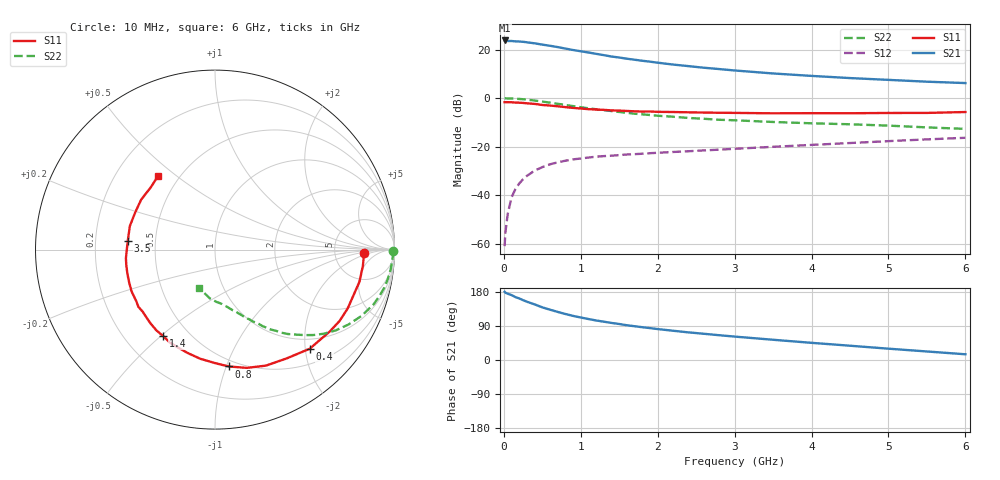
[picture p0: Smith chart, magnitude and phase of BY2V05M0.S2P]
! SIEMENS Small Signal Semiconductors
! BFY420
! Si NPN RF SIEGET Grounded Emitter Transistor in MICRO-X
! VCE = 2 V  IC = 5 mA
! Common Emitter S-Parameters:  October  1996
# GHz  S  MA  R  50
!  f  S11  S21  S12  S22
! GHz  MAG  ANG  MAG  ANG  MAG  ANG  MAG  ANG
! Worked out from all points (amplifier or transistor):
!   36 points, 10 MHz to 6 GHz, reference 50 ohm
!   highest |S21| = 23.8 dB at 10 MHz (marker M1)
!   |S21| within 3 dB of that: start of sweep to 743.9 MHz
!   unconditionally stable (mu >= 1): 3.149 GHz to end of sweep
!   at 250 MHz: K = 0.11, MSG = 28.3 dB, |S12| = -33.4 dB
!   at 1.4 GHz: K = 0.53, MSG = 20.4 dB, |S12| = -23.7 dB
!   at 6 GHz: K = 1.14, MAG = 9.0 dB, |S12| = -16.3 dB
!   S11 on the Smith chart (normalised r, x): 10 MHz: 10, -1; 400 MHz: 0.79, -2.09; 800 MHz: 0.45, -1.02; 1.4 GHz: 0.36, -0.51; 3.5 GHz: 0.34, +0.04; 6 GHz: 0.38, +0.43
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0.01  0.8283 -1.4  15.45 180.0  0.0009 110.8  0.9908 -0.5
0.02  0.8297 -2.6  15.36 177.6  0.0017 81.7  0.9938 -1.3
0.05  0.829 -6.2  15.06 174.9  0.0041 88.1  0.9894 -3.1
0.1  0.8247 -12.5  15.06 171.3  0.0091 85.3  0.985 -6.5
0.15  0.8129 -18.0  14.8 166.0  0.0134 78.6  0.9762 -9.8
0.2  0.8088 -23.9  14.7 162.5  0.0175 78.4  0.9666 -12.7
0.3  0.7855 -35.5  14.16 153.8  0.0252 71.8  0.9356 -18.9
0.4  0.7639 -46.3  13.49 146.8  0.0323 66.4  0.8966 -24.3
0.5  0.726 -56.6  12.68 138.9  0.0381 61.9  0.8528 -29.3
0.6  0.706 -66.3  12.02 132.8  0.0436 57.7  0.8103 -33.7
0.7  0.6826 -74.9  11.28 126.9  0.0478 54.3  0.7677 -37.6
0.8  0.6557 -83.3  10.51 121.4  0.0517 50.8  0.7257 -41.0
0.9  0.6316 -90.2  9.829 116.4  0.0551 48.2  0.6881 -43.8
1.1  0.596 -104.7  8.734 108.1  0.0601 44.4  0.6212 -49.2
1.4  0.5612 -121.1  7.213 97.8  0.0656 40.3  0.5443 -55.0
1.8  0.5309 -139.3  5.901 86.5  0.072 37.2  0.4655 -60.8
2.2  0.5199 -153.4  4.928 77.2  0.0782 35.6  0.4157 -65.8
2.8  0.502 -169.8  3.979 65.4  0.0874 34.1  0.36 -72.0
3.5  0.4886 174.5  3.232 53.4  0.0999 32.5  0.3244 -78.4
4.5  0.4905 154.9  2.598 37.7  0.1195 28.6  0.2907 -88.7
5.5  0.4982 136.0  2.188 22.5  0.1421 23.1  0.2508 -103.2
6  0.5196 127.4  2.05 15.1  0.1533 19.8  0.2336 -112.5
